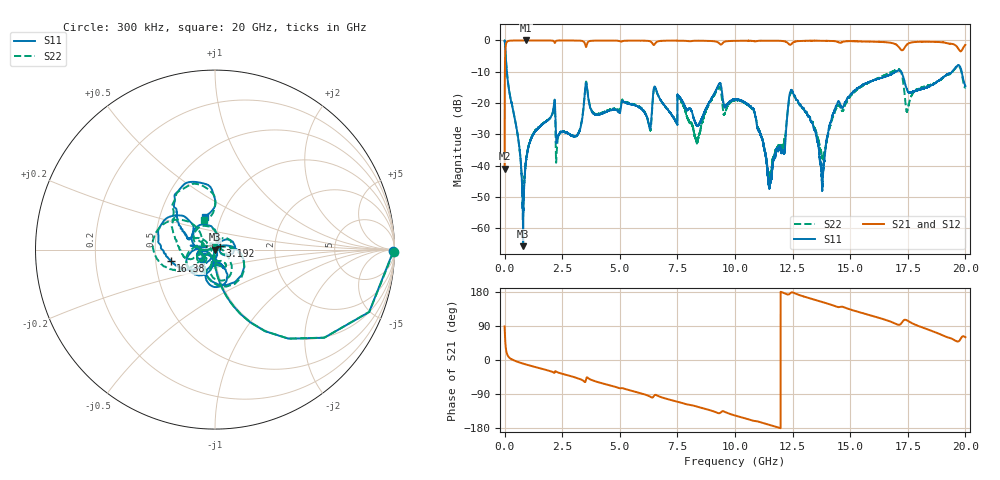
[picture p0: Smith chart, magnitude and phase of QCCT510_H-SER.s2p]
!{QCCT510}
!Johanson Technology Inc.
!www.johansontechnology.com
!Test Board Conditions:
!Substrate Type  RO4350B
!Substrate Thickness  20 mil
!Substrate Dk  3.66
!TL Type: GCPW
!TL Trace Width  34 mil
!TL Gap  10 mil
!Electrode orientation  Horizontal
!DUT TOPOLOGY	SERIES
!Mounting Pad LxW  26x52 mil
! Created Sat Jan  9 19:18:48 2021
# hz S ma R 50
! 2 Port Network Data from SP1.SP block
! freq  magS11  angS11  magS21  angS21  magS12  angS12  magS22  angS22
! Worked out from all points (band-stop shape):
!   20001 points, 300 kHz to 20 GHz, reference 50 ohm
!   highest |S21| = -0.01 dB at 935.3 MHz (marker M1); lowest = -40.9 dB at 300 kHz (marker M2)
!   |S21| within 3 dB of the highest: 33.2 MHz to 17.21 GHz (17.18 GHz wide, 199 % of centre); 17.29 GHz to 19.73 GHz (2.433 GHz wide, 13.1 % of centre)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
!   lowest |S11| = -65.7 dB at 805.3 MHz (marker M3), VSWR 1.00, Z = 50 + j0.0153 ohm
!   |S11| at or under -10 dB: 97.98 MHz to 16.95 GHz (16.85 GHz wide, 198 % of centre); 17.22 GHz to 19.42 GHz (2.196 GHz wide, 12 % of centre); 19.84 GHz to end of sweep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
!   |S22| runs from -55.0 to 0.0 dB; largest |S21 - S12| = 0.015
!   S11 on the Smith chart (normalised r, x): 300 kHz: open; 3.192 GHz: 1.05, +0.04; 16.38 GHz: 0.60, -0.08; 20 GHz: 0.84, +0.31
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300000  0.9933 -0.5  0.008994 88.7  0.009033 89.0  0.9951 -0.7
1.203e8  0.2608 -76.6  0.9645 13.6  0.9643 13.6  0.2617 -76.5
8.053e8  0.0005217 162.9  0.9975 -9.6  0.9993 -9.6  0.002174 153.6
9.353e8  0.01251 79.9  0.9994 -11.9  0.9975 -11.9  0.0129 86.8
2.1013e9  0.07448 46.3  0.9896 -32.1  0.9898 -32.1  0.0732 58.4
3.1923e9  0.03246 36.1  0.995 -48.5  0.9951 -48.4  0.03266 31.5
3.3343e9  0.04766 28.3  0.9872 -51.8  0.9874 -51.8  0.04907 20.3
3.5493e9  0.2079 -72.3  0.8027 -48.0  0.8033 -48.0  0.2157 -72.9
6.2823e9  0.04191 -156.6  0.9757 -95.6  0.9771 -95.5  0.04197 -163.3
6.6673e9  0.1332 -174.5  0.9694 -95.1  0.9695 -95.0  0.1314 179.6
8.3363e9  0.04391 -129.4  0.9896 -122.8  0.9892 -122.7  0.02407 60.3
1.00003e10  0.1142 -64.9  0.9834 -146.4  0.9856 -146.4  0.1107 -57.1
1.07953e10  0.08166 -75.0  0.9791 -160.4  0.9784 -160.3  0.0785 -85.5
1.15083e10  0.004927 18.5  0.9919 -171.3  0.9918 -171.3  0.007722 173.0
1.24343e10  0.1611 131.4  0.8673 177.8  0.8666 177.7  0.1503 135.0
1.33343e10  0.04965 69.7  0.9887 161.2  0.989 161.2  0.05004 78.4
1.37923e10  0.004612 -32.9  0.9901 152.9  0.9866 152.9  0.0135 133.7
1.44303e10  0.09666 -128.6  0.9555 140.5  0.9564 140.5  0.08603 -153.9
1.63793e10  0.2542 -165.8  0.9431 108.9  0.9397 108.7  0.2671 -155.8
1.66673e10  0.2762 -174.9  0.9274 102.9  0.9156 102.9  0.2987 -161.7
1.74853e10  0.1587 139.5  0.8711 104.0  0.8739 104.1  0.07746 -179.9
2e10  0.1883 108.4  0.8465 60.0  0.8407 60.2  0.1771 111.6
